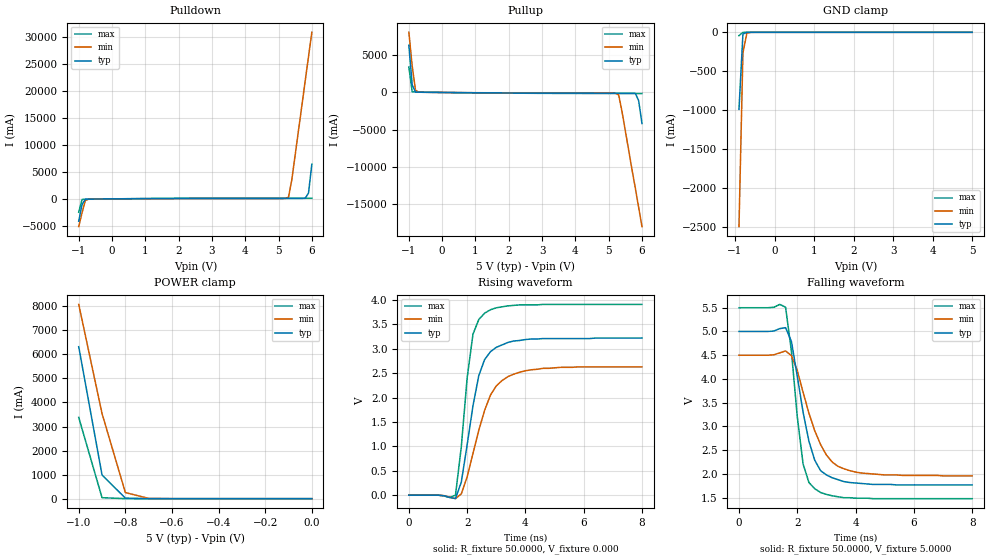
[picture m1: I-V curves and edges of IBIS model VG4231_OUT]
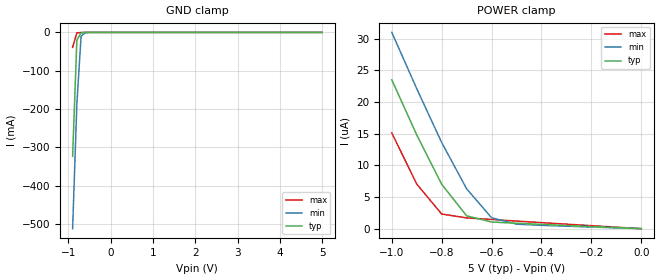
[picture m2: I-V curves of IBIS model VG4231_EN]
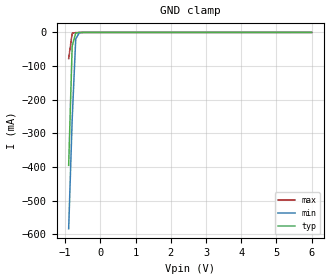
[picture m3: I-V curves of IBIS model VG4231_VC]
[IBIS ver]   2.1
[File name]   423acahf.ibs
[File Rev]   0.1
[Date]   March 23, 2005
[Copyright]   Copyright 2005, EPSONTOYOCOM Corp.
|   Component VG4231xxH
[Component]   VG4231xxH
[Manufacturer]   EPSONTOYOCOM Corp.
[Package]
| variable   typ   min   max
R_pkg   0.20   0.13   0.28
L_pkg   5.16nH   4.56nH   5.76nH
C_pkg   1.23pF   1.03pF   1.53pF
[Pin]  signal_name   model_name   R_pin   L_pin   C_pin
1   VC   VG4231_VC
2   NC   NC
3   GND   GND
4   OUT   VG4231_OUT
5   OE   VG4231_EN
6   VDD   POWER
| Models and submodels in the file (3): VG4231_OUT (3-state), VG4231_EN (Input), VG4231_VC (Input)
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|   Model VG4231_OUT
[Model]   VG4231_OUT
Model_type   3-state
Polarity   Non-Inverting
Enable   Active-High
C_comp   2.2010pF   2.2010pF   2.2010pF
[Temperature Range]   27.0000   85.0000   -40.0000
[Voltage Range]   5.0000V   4.5000V   5.5000V
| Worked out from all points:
|   slope of the pulldown table from 0 to 0.75 V, typ, clamps not added: 21.8 ohm
|   slope of the pullup table from 0 to 0.75 V, typ, clamps not added: 23.5 ohm
|   GND clamp passes 1 mA (typ) near -0.70 V on its own axis
|   POWER clamp passes 1 mA (typ) near -0.70 V on its own axis
|   rising waveform, R_fixture 50.0000, V_fixture 0.000: 20-80 % time 578ps typ, 794ps min, 404ps max; typ from 0 V to 3.22 V
|   falling waveform, R_fixture 50.0000, V_fixture 5.0000: 20-80 % time 618ps typ, 856ps min, 410ps max; typ from 5 V to 1.77 V
[Pulldown]
| voltage   I(typ)   I(min)   I(max)
-1V       -4.13A     -5.12A     -2.47A
-900mV    -1.03A     -2.53A     -103mA
-800mV    -62.6mA    -292mA     -55.7mA
-700mV    -36.8mA    -38.3mA    -48.7mA
5.1V      85.8mA     62.7mA     119mA
5.2V      85.9mA     72.8mA     119mA
5.3V      85.9mA     316mA      119mA
5.4V      86mA       3.6A       119mA
5.8V      108mA      21.8A      119mA
5.9V      1.07A      26.3A      119mA
6V        6.41A      30.8A      119mA
[Pullup]
| voltage   I(typ)   I(min)   I(max)
-1V       6.37A      8.12A      3.44A
-900mV    1.03A      3.58A      97.2mA
-800mV    60.7mA     286mA      51.1mA
-700mV    35.1mA     38.8mA     44.2mA
5.1V      -103mA     -78.6mA    -139mA
5.2V      -103mA     -89mA      -140mA
5.3V      -104mA     -339mA     -140mA
5.4V      -104mA     -2.57A     -140mA
5.7V      -105mA     -10.4A     -141mA
5.8V      -127mA     -12.9A     -142mA
5.9V      -1.09A     -15.5A     -142mA
6V        -4.19A     -18.1A     -142mA
[GND_clamp]
| voltage   I(typ)   I(min)   I(max)
-900mV    -988mA     -2.49A     -42.8mA
-800mV    -22.3mA    -261mA     -1.3mA
-700mV    -968uA     -10.8mA    -315uA
-500mV    -14.7uA    -62uA      -1.68uA
5V        113pA      95.8uA     93pA
[POWER_clamp]
| voltage   I(typ)   I(min)   I(max)
-1V       6.32A      8.08A      3.38A
-900mV    985mA      3.54A      40.6mA
-800mV    21.5mA     254mA      540uA
-700mV    770uA      10.7mA     43.6uA
-600mV    84.6uA     712uA      4.3uA
-500mV    10.8uA     95.8uA     259nA
-400mV    1.01uA     13.7uA     7.74nA
-300mV    59.4nA     1.55uA     282pA
-200mV    2.52nA     124nA      134pA
-100mV    191pA      7.24nA     127pA
0V        113pA      229pA      121pA
[Ramp]
| variable   typ   min   max
dV/dt_r   1.93/0.558n   1.58/0.784n   2.35/0.371n
dV/dt_f   1.94/0.596n   1.52/0.841n   2.41/0.396n
R_load = 50.0000
[Rising Waveform]
R_fixture = 50.0000
V_fixture = 0.000
V_fixture_min = 0.000
V_fixture_max = 0.000
| time   V(typ)   V(min)   V(max)
0s        2.41nV     12.3nV     1.29nV
1.6ns     -68.8mV    -71.5mV    434uV
1.8ns     267mV      26.1mV     993mV
2ns       1.03V      375mV      2.4V
2.2ns     1.83V      856mV      3.3V
2.4ns     2.45V      1.33V      3.6V
2.6ns     2.78V      1.74V      3.73V
3ns       3.03V      2.24V      3.84V
3.8ns     3.17V      2.52V      3.9V
8ns       3.22V      2.63V      3.91V
[Falling Waveform]
R_fixture = 50.0000
V_fixture = 5.0000
V_fixture_min = 4.5000
V_fixture_max = 5.5000
| time   V(typ)   V(min)   V(max)
0s        5V         4.5V       5.5V
1.6ns     5.08V      4.59V      5.51V
1.8ns     4.79V      4.49V      4.58V
2ns       4.06V      4.18V      3.21V
2.2ns     3.3V       3.72V      2.21V
2.4ns     2.69V      3.28V      1.82V
2.6ns     2.29V      2.91V      1.69V
3.2ns     1.92V      2.25V      1.54V
3.8ns     1.82V      2.07V      1.5V
8ns       1.77V      1.96V      1.48V
|   Model VG4231_EN
[Model]   VG4231_EN
Model_type   Input
Vinl =   1.0000V
Vinh =   4.0000V
C_comp   1.4070pF   1.4070pF   1.4070pF
[Temperature Range]   27.0000   85.0000   -40.0000
[Voltage Range]   5.0000V   4.5000V   5.5000V
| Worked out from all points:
|   GND clamp passes 1 mA (typ) near -0.70 V on its own axis
[GND_clamp]
| voltage   I(typ)   I(min)   I(max)
-900mV    -323mA     -512mA     -39mA
-800mV    -20.3mA    -187mA     -1.24mA
-700mV    -918uA     -9.88mA    -315uA
-600mV    -141uA     -601uA     -41.7uA
5V        27.5pA     712nA      25pA
[POWER_clamp]
| voltage   I(typ)   I(min)   I(max)
-1V       23.5uA     31uA       15.1uA
-900mV    14.8uA     22.1uA     7.04uA
-800mV    7.01uA     13.6uA     2.31uA
-700mV    2.02uA     6.29uA     1.7uA
-600mV    1.05uA     1.72uA     1.45uA
-500mV    851nA      712nA      1.2uA
-400mV    674nA      526nA      953nA
-300mV    501nA      388nA      709nA
-200mV    331nA      256nA      469nA
-100mV    164nA      126nA      233nA
0V        27.5pA     152pA      27.5pA
|   Model VG4231_VC
[Model]   VG4231_VC
Model_type   Input
Vinl =   1.000V
Vinh =   4.000V
C_comp   1.4070pF   1.4070pF   1.4070pF
[Temperature Range]   27.0000   85.0000   -40.0000
[Voltage Range]   5.0000V   4.5000V   5.5000V
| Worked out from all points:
|   GND clamp passes 1 mA (typ) near -0.65 V on its own axis
[GND_clamp]
| voltage   I(typ)   I(min)   I(max)
-900mV    -395mA     -583mA     -77.7mA
-800mV    -40.6mA    -257mA     -2.48mA
-700mV    -1.84mA    -19.7mA    -632uA
-600mV    -282uA     -1.2mA     -81.5uA
6V        50uA       42.9uA     60uA
